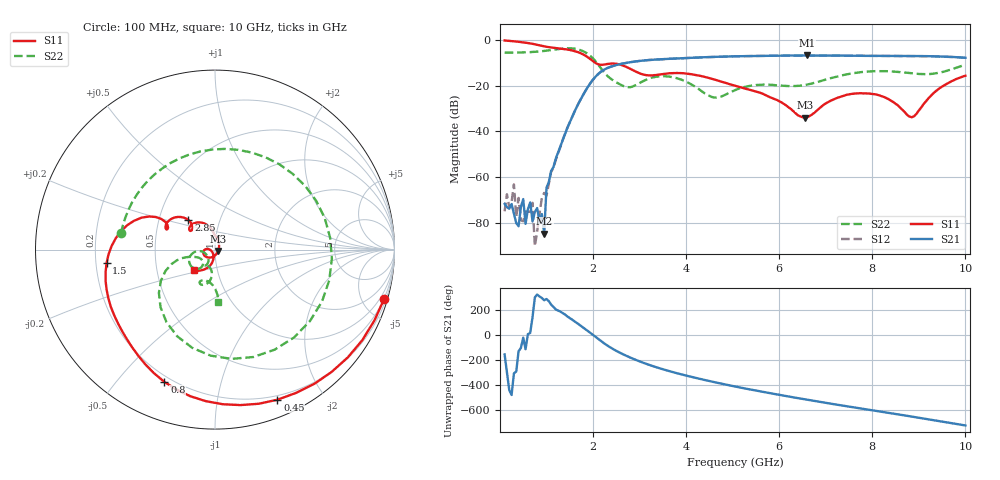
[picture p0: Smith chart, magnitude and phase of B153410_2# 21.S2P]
!  2-Port S-parameters saved by WinCal
! VAR MeasName=S-Parameters (CALIBRATED_DATA) read from VNA (N5245A)
! VAR MeasDate=2016-12-23 10:00:25
! VAR NAME=B153410_2# 21
! VAR FILENAME=B153410_2# 21.S2P
! VAR DATE=2016-12-23 10:00:25
! VAR PHYS_PORTS=1,2
# Hz S DB R 50
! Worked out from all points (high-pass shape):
!   199 points, 100 MHz to 10 GHz, reference 50 ohm
!   highest |S21| = -6.73 dB at 6.6 GHz (marker M1); lowest = -84.7 dB at 950 MHz (marker M2)
!   |S21| within 3 dB of the highest: 2.786 GHz to end of sweep
!   lowest |S11| = -33.9 dB at 6.55 GHz (marker M3), VSWR 1.04, Z = 51.9 - j0.809 ohm
!   |S11| at or under -10 dB: 2.052 GHz to end of sweep
!   |S22| runs from -25.2 to -3.6 dB; largest |S21 - S12| = 0.0022
!   S11 on the Smith chart (normalised r, x): 100 MHz: 0.46, -7.01; 450 MHz: 0.16, -1.49; 800 MHz: 0.17, -0.67; 1.5 GHz: 0.24, -0.06; 2.85 GHz: 0.71, +0.24; 10 GHz: 0.77, -0.18
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1e8  -0.16 -16.2  -71.75 -153.5  -74.97 89.1  -5.51 170.2
3e8  -0.52 -46.3  -75.96 54.3  -63.21 -20.1  -5.48 150.3
3.5e8  -0.63 -53.5  -80.14 68.5  -77.41 88.6  -5.48 145.0
4e8  -0.75 -60.5  -81.52 -128.4  -69.12 -159.5  -5.45 139.9
4.5e8  -0.86 -67.4  -73.06 -101.4  -78.91 149.0  -5.42 134.3
5.5e8  -1.13 -80.7  -80.48 -111.8  -74.99 -177.3  -5.36 123.1
6.5e8  -1.45 -93.4  -71.10 19.3  -75.11 -176.2  -5.27 111.1
7e8  -1.64 -99.6  -79.42 146.1  -71.26 -114.8  -5.21 104.8
8e8  -2.06 -111.0  -73.55 -32.0  -83.75 -28.1  -5.07 91.4
9.5e8  -2.73 -125.8  -84.73 -77.7  -66.93 -60.1  -4.76 69.4
1e9  -2.92 -130.2  -64.65 -68.0  -68.16 -86.4  -4.64 61.3
1.5e9  -4.31 -173.0  -36.00 139.0  -35.98 139.4  -3.58 -37.0
1.75e9  -5.89 164.5  -25.36 73.0  -25.31 72.8  -4.56 -92.3
2.85e9  -13.11 132.1  -9.53 172.8  -9.52 172.8  -20.33 -134.3
3.4e9  -15.15 143.1  -8.47 98.2  -8.45 98.1  -15.93 -141.5
5.05e9  -19.99 96.9  -7.10 -51.8  -7.12 -51.8  -21.92 -118.7
6.55e9  -33.91 -22.7  -6.76 -155.1  -6.76 -155.0  -19.72 -106.3
6.6e9  -33.83 -36.2  -6.73 -158.2  -6.75 -158.2  -19.49 -104.6
6.7e9  -32.66 -60.5  -6.74 -164.6  -6.75 -164.6  -19.01 -101.8
8.35e9  -25.88 176.9  -6.96 95.8  -6.95 95.9  -13.65 -113.7
8.85e9  -33.80 -141.7  -6.98 66.0  -6.98 66.1  -14.52 -113.5
1e10  -15.59 -135.7  -7.74 -5.3  -7.74 -5.3  -10.76 -86.3
